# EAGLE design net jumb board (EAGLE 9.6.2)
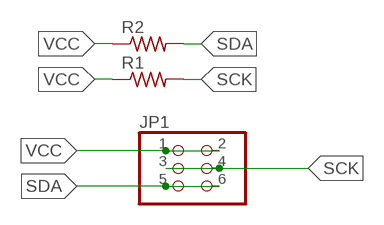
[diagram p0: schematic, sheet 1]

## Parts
JP1  PINHD-2X3-SMD  [2X03SMD]
R1  RES-US1206FAB  [R1206FAB]
R2  RES-US1206FAB  [R1206FAB]

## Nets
SCK: JP1.3 JP1.4 R1.2
SDA: JP1.5 JP1.6 R2.2
VCC: JP1.1 JP1.2 R1.1 R2.1

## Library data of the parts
JP1 = fab:PINHD-2X3-SMD: PIN HEADER
R1 R2 = fab:RES-US: Resistor (US Symbol)

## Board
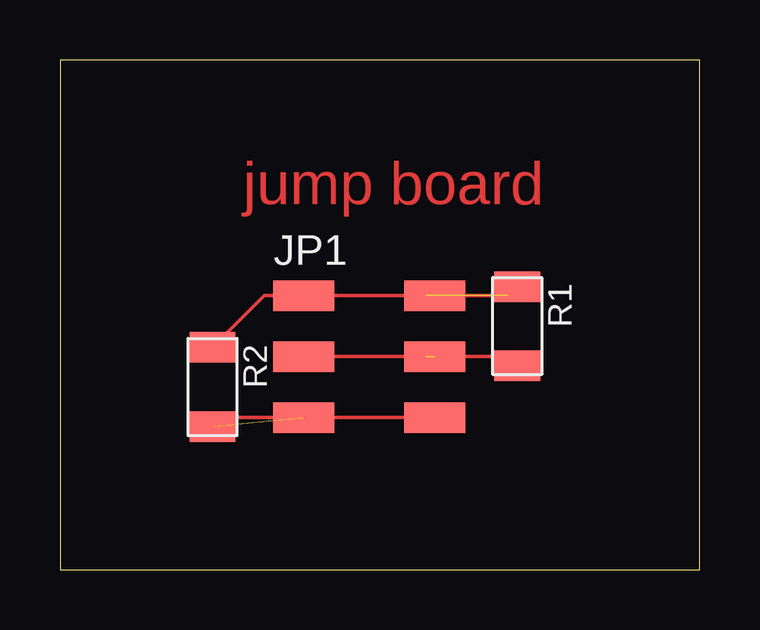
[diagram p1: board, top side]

Size 26.65 x 21.26 mm. Coordinates in mm from the lower left corner, seen from the top.
Outline: 0,0 26.65,0 26.65,21.26 0,21.26 0,0
Copper layers (1*16): Top 0.035mm / dielectric 1.5mm / Bottom 0.035mm
Design rules "default *": minimum track width 6mil, minimum drill 0.35mm, track to track 19mil, track to pad 19mil, pad to pad 6mil, via to via 6mil, smd to smd 6mil, copper to edge 40mil, drill to drill 6mil, minimum pad ring 10mil, minimum via ring 8mil, stop-mask expansion 4mil, vias tented up to drill 0mil, thermal gap 10mil

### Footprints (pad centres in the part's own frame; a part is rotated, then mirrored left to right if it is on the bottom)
2X03SMD = smd 2.54 x 1.27: 1 -2.54,2.54; 2 2.92,2.54; 3 -2.54,0; 4 2.92,0; 5 -2.54,-2.54; 6 2.92,-2.54
R1206FAB = smd 1.27 x 1.905: 1 -1.651,0; 2 1.651,0

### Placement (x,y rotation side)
JP1  12.7,8.89 0 top
R1  19.05,10.16 270 top
R2  6.35,7.62 270 top

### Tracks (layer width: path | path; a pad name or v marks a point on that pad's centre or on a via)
SCK  (1 unrouted)
  Top 0.152: R1.2 18.67,8.89 JP1.4 | JP1.3 15.24,8.89
SDA  (1 unrouted)
  Top 0.152: R2.2 6.73,6.35 JP1.6
VCC  (2 unrouted)
  Top 0.152: R2.1 8.51,11.43 JP1.1 15.24,11.43 | R1.1 18.67,11.43 JP1.2

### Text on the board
Top: jump board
